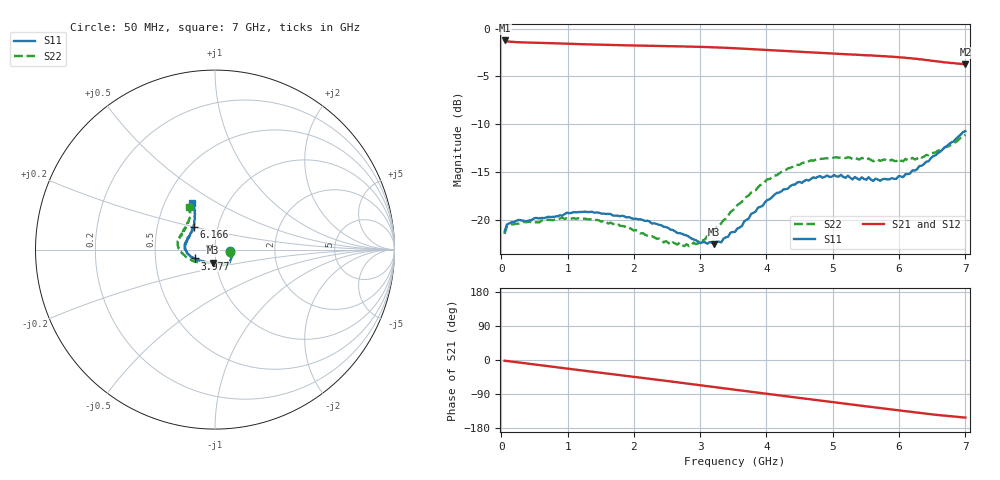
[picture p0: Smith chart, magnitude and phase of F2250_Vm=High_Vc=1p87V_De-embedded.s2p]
! Integrated Device Technology
! Corporate Headquarters
! 6024 Silver Creek Valley Road
! San Jose, CA 95138  USA
! Phone:  1-408-284-8200
! Toll Free:  1-800-223-1366
! Webpage:  http://www.idt.com/
! Timing and RF Division
! 515 Groton Road, Suite 102
! Westford, MA 01886-6024
! Device:  F2250
! Description: Voltage Variable RF Attenuator
! Frequency:  50.0 -  6000.00 MHz
! Package:  3x3 mm Thin QFN Plastic Package: 16 pin
! Ports:  2 RF, 3 DC
!  Pin  1  = GND
!  Pin  2  = NC
!  Pin  3  = RF1  = Port 1
!  Pin  4  = NC
!  Pin  5  = GND
!  Pin  6  = GND
!  Pin  7  = GND
!  Pin  8  = GND
!  Pin  9  = NC
!  Pin 10  = RF2  = Port 2
!  Pin 11  = NC
!  Pin 12  = GND
!  Pin 13  = GND
!  Pin 14  = VCNTRL
!  Pin 15  = VDD
!  Pin 16  = VMODE
! Vcntrl:  1.870 Volts
! Vmode:  +3.300 Volts
! Vdd:  +3.30  Volts
! Current:  1.324 mA
! Data:  The device was measured on a the F2250 evaluation board which has
!  individual transmission lines to the RF pins.  Data was collected
!  using a calibrated network analyzer.  The evaluation board was
!  de-embedded using a TRL calibration technique.
!  The reference plane is the edge of the package pin.
! Misc:  SN 10
!  Action Tracker AT0258
! Date Measured:  2014-11-26
! Date:  2015-10-15  MJV
! Note:
!  Integrated Device Technology supplies this data as a sample of measured
!  data at the package pin for this product.  Your particular data for this
!  product may vary.
!  Data was taken at 25 degrees C.
!  Integrated Device Technology reserves the right to change this data at anytime.
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# GHz S dB R 50
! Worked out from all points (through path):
!   201 points, 50 MHz to 7 GHz, reference 50 ohm
!   highest |S21| = -1.23 dB at 50 MHz (marker M1); lowest = -3.7 dB at 7 GHz (marker M2)
!   group delay of S21, straight-line fit = 61.1 ps
!   lowest |S11| = -22.6 dB at 3.212 GHz (marker M3), VSWR 1.16, Z = 48.4 - j7.16 ohm
!   |S11| at or under -10 dB: start of sweep to end of sweep
!   |S22| runs from -22.8 to -11.1 dB; largest |S21 - S12| = 0.0019
!   S11 on the Smith chart (normalised r, x): 50 MHz: 1.19, -0.02; 3.977 GHz: 0.79, -0.08; 6.166 GHz: 0.77, +0.20; 7 GHz: 0.68, +0.39
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0.05  -21.24 -6.4  -1.23 -1.8  -1.23 -1.8  -21.50 -7.5
0.08475  -20.50 -6.2  -1.32 -2.5  -1.32 -2.5  -20.68 -7.0
0.1195  -20.38 -6.8  -1.36 -3.3  -1.36 -3.3  -20.51 -6.9
0.71025  -19.69 -29.7  -1.51 -16.5  -1.51 -16.5  -19.99 -33.5
1.2315  -19.19 -45.1  -1.63 -27.9  -1.63 -27.9  -19.89 -53.4
1.75275  -19.57 -52.1  -1.72 -39.1  -1.72 -39.1  -20.41 -63.1
2.37825  -20.54 -54.4  -1.81 -52.6  -1.81 -52.7  -21.98 -71.5
2.552  -21.04 -58.1  -1.83 -56.5  -1.83 -56.5  -22.61 -78.0
2.691  -21.40 -63.3  -1.85 -59.6  -1.85 -59.6  -22.39 -84.2
2.83  -21.79 -68.4  -1.88 -62.7  -1.87 -62.7  -22.77 -92.8
3.07325  -22.37 -84.6  -1.92 -68.2  -1.92 -68.2  -22.04 -111.0
3.21225  -22.56 -98.8  -1.95 -71.3  -1.95 -71.4  -21.09 -122.3
3.525  -21.28 -127.5  -2.04 -78.4  -2.05 -78.5  -18.81 -141.0
3.97675  -18.19 -156.3  -2.21 -88.6  -2.22 -88.7  -16.01 -162.1
4.4285  -16.32 -171.3  -2.39 -98.6  -2.40 -98.6  -14.27 -176.7
4.7065  -15.56 -179.5  -2.49 -104.7  -2.49 -104.7  -13.82 176.9
5.054  -15.47 172.0  -2.62 -112.4  -2.62 -112.4  -13.45 169.2
5.61  -15.95 155.0  -2.81 -124.5  -2.81 -124.6  -13.88 156.8
5.85325  -15.77 144.9  -2.92 -129.8  -2.92 -129.9  -13.85 149.6
6.166  -15.16 132.7  -3.09 -136.7  -3.09 -136.8  -13.74 141.0
6.54825  -13.26 121.8  -3.39 -144.5  -3.39 -144.7  -12.97 128.7
7  -10.72 115.7  -3.72 -152.0  -3.73 -152.1  -11.12 122.1
